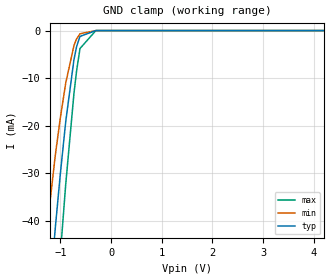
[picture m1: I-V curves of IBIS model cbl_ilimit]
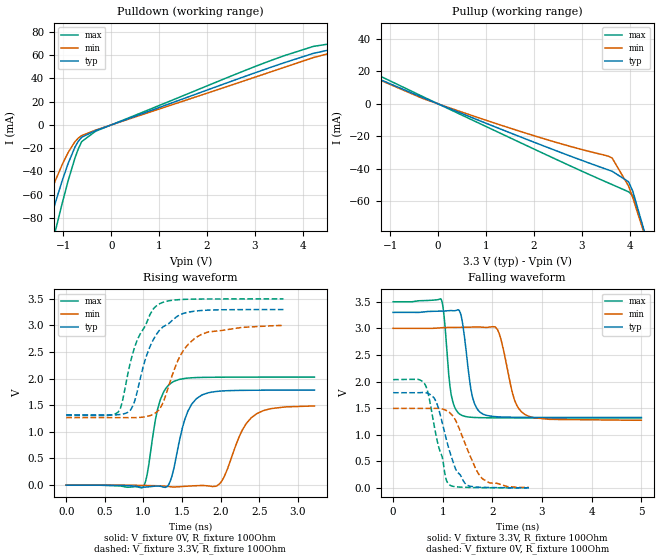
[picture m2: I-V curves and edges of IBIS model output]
|Texas Instruments Incorporated
| THUNDERBOLT BUS POWER BUCK/BOOST
| Marketing part#   Digital Voltage Range   Package-type   #pins
| TPS65980   2.9V-3.5V   QFN   24
[IBIS Ver]   4.1
[File name]   tps65980.ibs
[File Rev]   1.0
[Date]   4/3/2014
[Source]
| Texas Instruments Incorporated.
| Analog-eLab Design Center, HPA
| 12500 TI Blvd
| Dallas, TX -75243
[Notes]   Revision History:
| Rev 1.0: 4/3/2014
| - Initial version of the model
| - Model generated from simulations in TISPICE
| - Model matched to SPICE simulation
| - C_comp although listed in numerical order of value are
|   obtained from varying PVT conditions. For PVT conditions for
|   each specific value refer the buffer description under
|   respective [Model]. IBIS model user is responsible for using
|   appropriate C_comp to simulate for Signal Integrity.
[Disclaimer]
| This model is designed as an aid for customers of Texas Instruments.
| TI and its licensors and suppliers make no warranties, either expressed
| or implied, with respect to this  model, including the warranties of
| merchantability or fitness for a particular purpose. The model is
| provided solely on an "as is" basis. The entire risk as to its quality
| and performance is with the customer.
[Copyright]
(C) Copyright 2014 Texas Instruments Incorporated.All rights reserved.
|   TPS65980RHF
[Component]   TPS65980RHF
[Manufacturer]   TI
[Package]   |24 QFN  -  RHF package
|   typ   min   max
R_pkg   0.01297   0.01260   0.01345
L_pkg   0.82973nH   0.77866nH   0.93764nH
C_pkg   0.15695pF   0.14559pF   0.16337pF
[Pin]  signal_name   model_name   R_pin   L_pin   C_pin
1   SS   nc   0.01308   0.91851nH  0.13976pF
2   GND   gnd   0.01316   0.81769nH  0.16266pF
3   GND   gnd   0.00452   0.54711nH  0.20963pF
4   GND   gnd   0.01298   0.91275nH  0.15535pF
5   HV_OK   output   0.01309   0.81316nH  0.16337pF
6   RESET_N   output   0.01345   0.93764nH  0.15860pF
7   CBL_OUT   power   0.00486   0.60152nH  0.20492pF
8   CBL_ILIMIT   cbl_ilimit   0.01275   0.78945nH  0.14559pF
9   DEV_EN   dev_enz   0.01260   0.77866nH  0.16024pF
10   GND   gnd   0.01347   0.83210nH  0.16572pF
11   TBT_OUT   power   0.00703   0.62443nH  0.20571pF
12   TBT_OUT   power   0.00574   0.76249nH  0.22827pF
13   DEV_OUT   power   0.00664   0.61849nH  0.17411pF
14   DEV_OUT   power   0.00664   0.56385nH  0.19983pF
15   CPP   nc   0.00723   0.66476nH  0.19603pF
16   CPN   nc   0.00730   0.70731nH  0.19383pF
17   PGND   gnd   0.00668   0.60511nH  0.19063pF
18   PGND   gnd   0.00661   0.62390nH  0.18603pF
19   SW   nc   0.00837   0.75823nH  0.20152pF
20   SW   nc   0.00694   0.61921nH  0.18313pF
21   BOOT   nc   0.01317   0.81370nH  0.16446pF
22   TBT_IN   power   0.00665   0.56826nH  0.20119pF
23   TBT_IN   power   0.00456   0.57004nH  0.21856pF
24   COMP   nc   0.01302   0.91193nH  0.13992pF
| Models and submodels in the file (3): cbl_ilimit (Input), dev_enz (Input), output (Output)
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|   cbl_ilimit Model
[Model]   cbl_ilimit
Model_type   Input
Vinl = 0.6
Vinh = 2.6
|   typ   min   max
|   (nom PVT)   (fast PVT)   (slow PVT)
C_comp   6.470e-13   4.378e-13   8.599e-13
| Where nom  PVT is Nominal Process, 3V, 27C
|   Fast PVT is Strong Process,  3.1V, -40C
|   Slow PVT is Weak Process,   2.9V, 125C
[Voltage Range]   3   2.9   3.1
|Junction Temperature
[Temperature Range]   27   125   -40
[Power Clamp Reference]   3   2.9   3.1
[GND Clamp Reference]   0   0   0
[GND Clamp]
|   Voltage   I(typ)   I(min)   I(max)
-3V       -1.155A    -317.4mA   -1.861A
-1.434V   -83.95mA   -57.32mA   -113.7mA
-1.101V   -41.39mA   -26.17mA   -61.64mA
-1.002V   -30.14mA   -18.37mA   -47.11mA
-895.1mV  -19.14mA   -11.03mA   -32.28mA
-732.2mV  -6.069mA   -3.131mA   -13.18mA
-681mV    -3.408mA   -1.741mA   -8.504mA
-613mV    -1.225mA   -671.7uA   -3.767mA
-300.1mV  -351.9nA   -924.1nA   -496.4nA
6V        0A         0A         0A
[POWER Clamp]
|   Voltage   I(typ)   I(min)   I(max)
-3V       0A         0A         0A
0V        0A         0A         0A
6V        0A         0A         0A
|   output Model
[Model]   output
Model_type   Output
Polarity   Non-Inverting
Vmeas = 1.65
Vref = 0
Cref = 10pF
Rref = 150
|   typ   min   max
|   (nom PVT)   (fast PVT)   (slow PVT)
C_comp   8.663e-13   5.838e-13   1.087e-12
| Where nom  PVT is Nominal Process, 3.3V, 27C
|   Fast PVT is Strong Process,  3.5V, -40C
|   Slow PVT is Weak Process,   3V, 125C
[Voltage Range]   3.3   3   3.5
|Junction Temperature
[Temperature Range]   27   125   -40
[Pullup Reference]   3.3   3   3.5
[Pulldown Reference]   0   0   0
[Power Clamp Reference]   3.3   3   3.5
[GND Clamp Reference]   0   0   0
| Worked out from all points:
|   slope of the pulldown table from 0 to 0.495 V, typ, clamps not added: 66.7 ohm
|   slope of the pullup table from 0 to 0.495 V, typ, clamps not added: 83.4 ohm
|   falling waveform, V_fixture 3.3V, R_fixture 100Ohm: 20-80 % time 168ps typ, 253ps min, 127ps max; typ from 3.3 V to 1.32 V
|   rising waveform, V_fixture 0V, R_fixture 100Ohm: 20-80 % time 190ps typ, 263ps min, 153ps max; typ from 0 V to 1.79 V
|   rising waveform, V_fixture 3.3V, R_fixture 100Ohm: 20-80 % time 292ps typ, 314ps min, 292ps max; typ from 1.32 V to 3.3 V
|   falling waveform, V_fixture 0V, R_fixture 100Ohm: 20-80 % time 323ps typ, 399ps min, 282ps max; typ from 1.79 V to 0.002 V
[Pulldown]
|   Voltage   I(typ)   I(min)   I(max)
-3.3V     -1.248A    -672.2mA   -1.686A
-1.887V   -174.8mA   -132.3mA   -217.7mA
-1.449V   -107.6mA   -78.73mA   -140.3mA
-1.169V   -67.11mA   -48.03mA   -91.51mA
-900.9mV  -33.2mA    -23.75mA   -48.1mA
-759mV    -19.17mA   -14.49mA   -28.58mA
-689.7mV  -14.14mA   -11.4mA    -20.75mA
-619mV    -10.64mA   -9.233mA   -14.44mA
-330mV    -4.952mA   -4.534mA   -5.507mA
2.963V    44.33mA    40.6mA     49.68mA
4.218V    61.62mA    57.97mA    67.63mA
6.6V      83.04mA    84.16mA    82.88mA
[Pullup]
|   Voltage   I(typ)   I(min)   I(max)
-3.3V     41.01mA    41.16mA    46.69mA
-330mV    3.985mA    3.418mA    4.622mA
1.812V    -21.4mA    -17.84mA   -25.18mA
2.721V    -31.7mA    -25.85mA   -37.65mA
3.603V    -41.16mA   -32.87mA   -49.28mA
3.633V    -41.47mA   -33.39mA   -49.66mA
3.972V    -47.9mA    -50.44mA   -54.07mA
4.064V    -53.89mA   -57.85mA   -56.64mA
4.31V     -79.09mA   -80.64mA   -79.46mA
6.6V      -1.257A    -1.048A    -1.429A
[Ramp]
R_load = 100
|   typ   min   max
dV/dt_r   1.07218/1.88363e-10   0.895423/2.63337e-10   1.21856/1.51599e-10
dV/dt_f   1.18542/1.67131e-10   1.03665/2.5001e-10   1.31093/1.27105e-10
[Falling Waveform]
V_fixture = 3.3V
V_fixture_min = 3V
V_fixture_max = 3.5V
R_fixture = 100Ohm
|   Time   V(typ)   V(min)   V(max)
0s        3.3V       3V         3.5V
968ps     3.324V     3.011V     3.546V
1.17ns    3.334V     3.017V     1.754V
1.384ns   3.177V     3.02V      1.365V
1.596ns   1.719V     3.024V     1.327V
1.808ns   1.389V     3.021V     1.32V
2.104ns   1.337V     2.976V     1.317V
2.442ns   1.329V     1.663V     1.316V
2.652ns   1.327V     1.382V     1.316V
5ns       1.324V     1.272V     1.315V
[Rising Waveform]
V_fixture = 0V
V_fixture_min = 0V
V_fixture_max = 0V
R_fixture = 100Ohm
|   Time   V(typ)   V(min)   V(max)
0s        381.8pV    6.919nV    229.3pV
992ps     -40.4mV    -6.746mV   -42.26mV
1.216ns   -20.91mV   -14.12mV   1.596V
1.4ns     356.5mV    -35.4mV    1.953V
1.574ns   1.385V     -19.44mV   2.011V
1.754ns   1.691V     -7.272mV   2.024V
2.004ns   1.768V     55.69mV    2.028V
2.282ns   1.781V     1.04V      2.029V
2.462ns   1.783V     1.339V     2.03V
3.214ns   1.786V     1.485V     2.031V
[Rising Waveform]
V_fixture = 3.3V
V_fixture_min = 3V
V_fixture_max = 3.5V
R_fixture = 100Ohm
|   Time   V(typ)   V(min)   V(max)
0s        1.32V      1.268V     1.309V
674ps     1.323V     1.268V     1.375V
728ps     1.334V     1.268V     1.581V
822ps     1.39V      1.268V     2.253V
918ps     1.75V      1.269V     2.72V
1.044ns   2.452V     1.291V     3.062V
1.21ns    2.914V     1.428V     3.409V
1.466ns   3.195V     2.403V     3.486V
1.688ns   3.273V     2.78V      3.496V
2.812ns   3.299V     3V         3.5V
[Falling Waveform]
V_fixture = 0V
V_fixture_min = 0V
V_fixture_max = 0V
R_fixture = 100Ohm
|   Time   V(typ)   V(min)   V(max)
0s        1.79V      1.495V     2.036V
652ps     1.791V     1.495V     1.93V
882ps     1.586V     1.496V     911.3mV
994ps     1.209V     1.484V     559.1mV
1.064ns   943.5mV    1.459V     174mV
1.132ns   709.5mV    1.42V      59.51mV
1.256ns   360.9mV    1.274V     22.37mV
1.442ns   93.3mV     851.4mV    11.25mV
1.808ns   10.6mV     166.5mV    4.221mV
2.736ns   2.412mV    11.07mV    1.413mV
